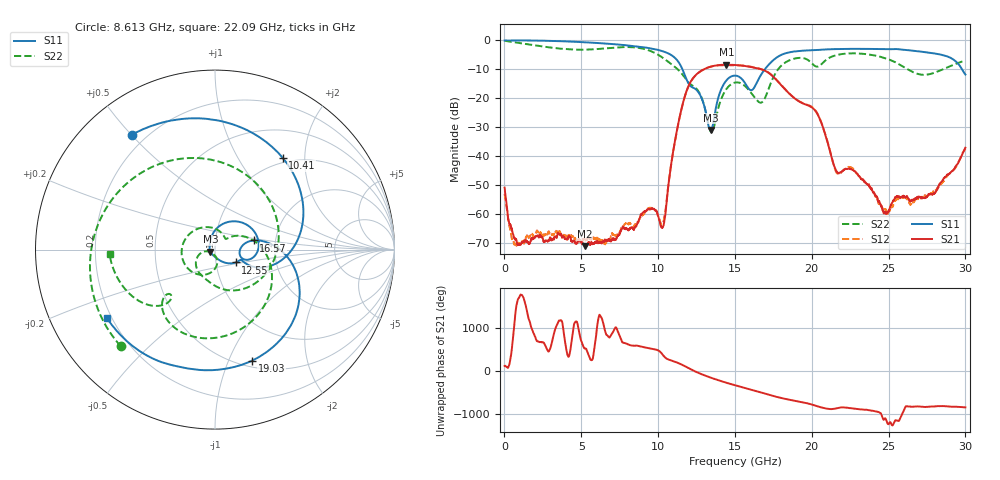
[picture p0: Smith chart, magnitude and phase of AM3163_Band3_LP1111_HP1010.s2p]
!Agilent Technologies,E8364B,MY43040894,A.07.50.67
!Agilent E8364B: A.07.50.67
!Date: Thursday, August 20, 2020 12:18:25
!Correction: S11(Full 2 Port(1,2))
!S21(Full 2 Port(1,2))
!S12(Full 2 Port(1,2))
!S22(Full 2 Port(1,2))
!S2P File: Measurements: S11, S21, S12, S22:
# Hz S  dB  R 50
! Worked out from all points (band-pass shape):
!   3201 points, 10 MHz to 30 GHz, reference 50 ohm
!   highest |S21| = -8.39 dB at 14.44 GHz (marker M1); lowest = -71.2 dB at 5.221 GHz (marker M2)
!   |S21| within 3 dB of the highest: 12.57 GHz to 17.24 GHz (4.67 GHz wide, 31.3 % of centre)
!   lowest |S11| = -31.0 dB at 13.41 GHz (marker M3), VSWR 1.06, Z = 47.5 - j1.14 ohm
!   |S11| at or under -10 dB: 11.59 GHz to 16.94 GHz (5.359 GHz wide, 37.6 % of centre); 29.78 GHz to end of sweep
!   |S22| runs from -31.7 to -0.1 dB; largest |S21 - S12| = 0.011
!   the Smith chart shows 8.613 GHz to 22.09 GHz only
!   S11 on the Smith chart (normalised r, x): 8.613 GHz: 0.15, +0.50; 10.41 GHz: 0.92, +1.57; 12.55 GHz: 1.24, -0.18; 16.57 GHz: 1.54, +0.17; 19.03 GHz: 0.57, -1.22; 22.09 GHz: 0.18, -0.28
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1e7  -0.01 -2.1  -50.97 118.8  -53.11 107.9  -0.12 -5.0
5.723125e8  -0.01 -15.4  -67.10 107.3  -69.34 171.3  -0.57 -39.8
1.247088e9  -0.00 -33.7  -69.58 -100.9  -70.14 20.7  -1.12 -82.3
2.662241e9  -0.10 -71.8  -69.44 -130.3  -67.27 -63.5  -2.22 -162.7
5.014581e9  -0.57 -133.1  -69.70 -34.1  -69.10 65.3  -3.21 73.5
5.220762e9  -0.63 -138.5  -71.21 167.6  -68.81 172.8  -3.19 62.3
6.748378e9  -1.14 -178.9  -69.06 82.0  -69.59 -105.4  -2.65 -22.9
8.613381e9  -2.05 125.8  -63.69 -129.0  -63.09 154.7  -2.48 -134.3
1.000979e10  -3.30 72.8  -60.83 119.5  -60.83 123.9  -4.99 120.5
1.041278e10  -3.94 53.7  -62.20 -27.1  -60.87 119.7  -6.41 81.2
1.146243e10  -8.64 -9.9  -25.06 162.4  -25.16 162.4  -10.98 -46.4
1.254957e10  -17.39 -32.0  -11.48 -31.1  -11.55 -30.4  -17.03 -138.0
1.341178e10  -31.02 -154.7  -9.09 -152.0  -9.08 -152.0  -31.42 -137.6
1.444269e10  -13.84 49.9  -8.39 87.8  -8.57 88.2  -16.85 -107.8
1.5005e10  -12.16 11.8  -8.49 29.3  -8.60 30.8  -14.58 -152.8
1.65701e10  -13.09 13.3  -9.75 -125.0  -9.72 -124.5  -21.36 50.2
1.902553e10  -3.71 -71.5  -20.59 19.6  -20.54 20.1  -6.12 -92.3
2.000958e10  -3.39 -99.2  -23.18 -59.2  -22.99 -58.8  -7.92 -136.2
2.209014e10  -2.93 -147.7  -44.86 -126.2  -44.65 -127.7  -4.62 -177.4
2.500479e10  -3.01 144.9  -59.16 -156.0  -59.36 -4.3  -6.55 68.2
2.741336e10  -4.08 77.5  -54.40 -115.4  -53.66 -115.3  -11.88 -89.0
3e10  -11.80 -28.6  -37.11 -126.9  -37.47 -124.2  -6.92 131.0
